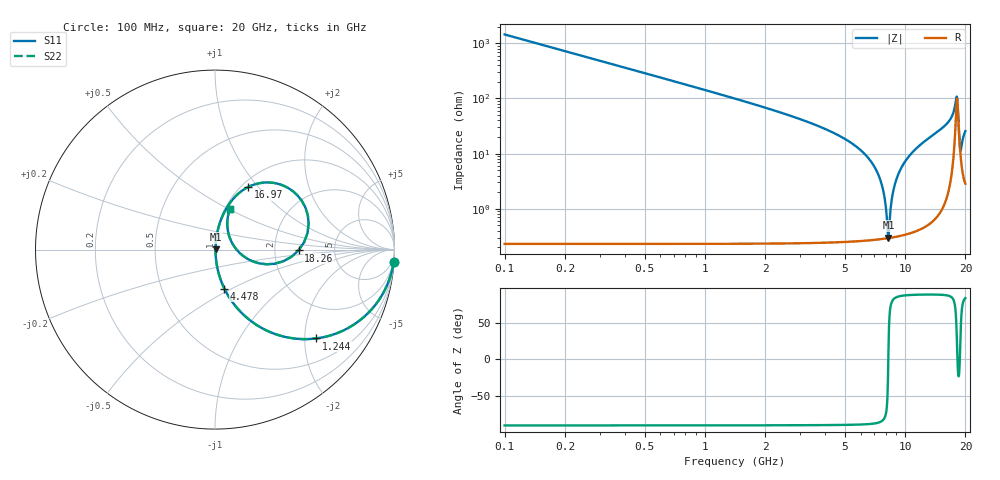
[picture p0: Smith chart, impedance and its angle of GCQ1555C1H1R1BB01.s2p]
!Murata Part Number: GCQ1555C1H1R1BB01
!These Parameters are Measured in Series Mode Connection
!Data Generated on Mar 13, 2026
!  o--ll--o
!Port1  Port2
!  o------o
!Operation Temp=25[degC], DC Bias Voltage=0[V]
!Freq. Start=100[MHz] Stop=20[GHz] 401[Steps]
# Hz S RI R 50
!Freq.(Hz) S11(Real) S11(Imag) S21(Real) S21(Imag) S12(Real) S12(Imag) S22(Real) S22(Imag)
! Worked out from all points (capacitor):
!   401 points, 100 MHz to 20 GHz, reference 50 ohm
!   read as one part in series: C = 1.1 pF near 199.5 MHz
!   lowest |Z| = 301 mohm at 8.259 GHz (marker M1)
!   series resonance near 8.244 GHz, so ESL is about 340 pH
!   S11 on the Smith chart (normalised r, x): 100 MHz: 1, -29; 1.244 GHz: 1.00, -2.27; 4.478 GHz: 1.00, -0.46; 16.97 GHz: 1.07, +0.88; 18.26 GHz: 2.74, -0.03; 20 GHz: 1.06, +0.51
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1e8  0.9952 -0.0688  0.00477 0.0688  0.00477 0.0688  0.9952 -0.0688
2.99e8  0.9589 -0.1984  0.0411 0.1984  0.0411 0.1984  0.9589 -0.1984
4.98e8  0.8932 -0.3084  0.1068 0.3084  0.1068 0.3084  0.8932 -0.3084
1.24425e9  0.5638 -0.4949  0.4362 0.4949  0.4362 0.4949  0.5638 -0.4949
2.1895e9  0.2755 -0.4449  0.7245 0.4449  0.7245 0.4449  0.2755 -0.4449
3.43325e9  0.1109 -0.3106  0.8891 0.3106  0.8891 0.3106  0.1109 -0.3106
4.478e9  0.0523 -0.2173  0.9477 0.2173  0.9477 0.2173  0.0523 -0.2173
6.7665e9  0.0077 -0.0706  0.9923 0.0706  0.9923 0.0706  0.0077 -0.0706
7.71175e9  0.00341 -0.024  0.9966 0.024  0.9966 0.024  0.00341 -0.024
8.259e9  0.00293 0.000646  0.9971 -0.000646  0.9971 -0.000646  0.00293 0.000646
8.5575e9  0.00317 0.0135  0.9968 -0.0135  0.9968 -0.0135  0.00317 0.0135
8.856e9  0.00374 0.026  0.9963 -0.026  0.9963 -0.026  0.00374 0.026
1.005e10  0.00877 0.0731  0.9912 -0.0731  0.9912 -0.0731  0.00877 0.0731
1.338325e10  0.0437 0.1913  0.9563 -0.1913  0.9563 -0.1913  0.0437 0.1913
1.67165e10  0.1573 0.3327  0.8427 -0.3327  0.8427 -0.3327  0.1573 0.3327
1.696525e10  0.1836 0.3481  0.8164 -0.3481  0.8164 -0.3481  0.1836 0.3481
1.776125e10  0.3879 0.3534  0.6121 -0.3534  0.6121 -0.3534  0.3879 0.3534
1.805975e10  0.5171 0.1916  0.4829 -0.1916  0.4829 -0.1916  0.5171 0.1916
1.825875e10  0.4654 -0.00444  0.5346 0.00444  0.5346 0.00444  0.4654 -0.00444
1.85075e10  0.2476 -0.077  0.7524 0.077  0.7524 0.077  0.2476 -0.077
1.89055e10  0.0898 0.048  0.9102 -0.048  0.9102 -0.048  0.0898 0.048
2e10  0.0839 0.227  0.9161 -0.227  0.9161 -0.227  0.0839 0.227
